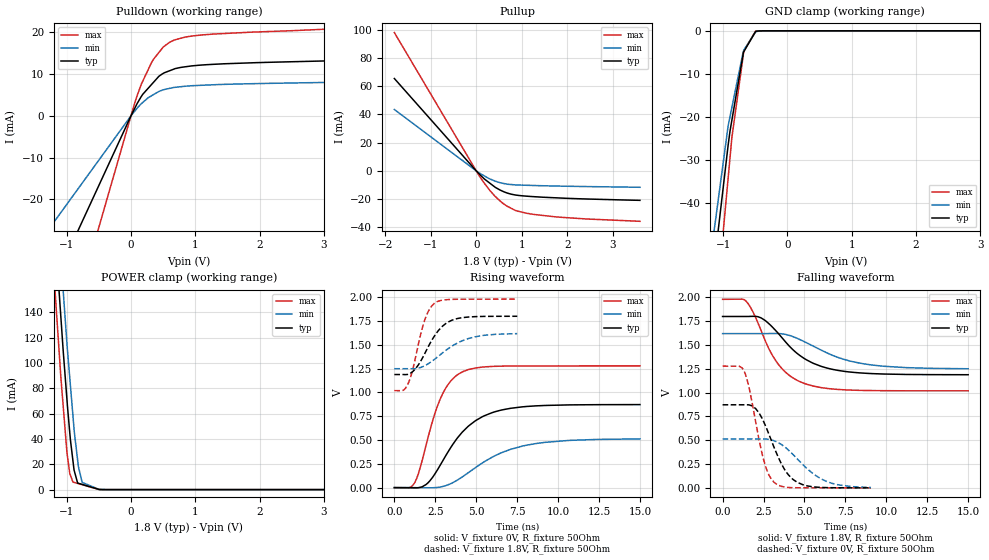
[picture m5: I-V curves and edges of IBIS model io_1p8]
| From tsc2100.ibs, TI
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|   io_1p8 Model
[Model]   io_1p8
Model_type   I/O
Polarity   Non-Inverting
Enable   Active-Low
Vinl = 0.54
Vinh = 1.26
Vmeas = 0.9
Vref = 0.9
Cref = 10pF
Rref = 50
|   typ   min   max
|   (nom PVT)   (fast PVT)   (slow PVT)
|C_comp from frequency sweep method (F=13MHz)
|Average
|C_comp   3.038e-12   2.861e-12   3.135e-12
|ON state : BUFFER OUTPUT TURNED HIGH
|C_comp   4.296e-12   3.958e-12   4.472e-12
|OFF state: BUFFER IN HIGH IMPEDANCE
|C_comp   1.781e-12   1.764e-12   1.798e-12
|C_comp from LC tank measurement(L=1nH)
|Average
|Resonant Frequency(Hz)   4.230e+09   4.260e+09   4.200e+09
C_comp   1.419e-12   1.398e-12   1.440e-12
|ON state : BUFFER OUTPUT TURNED HIGH
|Resonant Frequency(Hz)   4.150e+09   4.180e+09   4.100e+09
|C_comp   1.472e-12   1.451e-12   1.508e-12
|OFF state: BUFFER IN HIGH IMPEDANCE
|Resonant Frequency(Hz)   4.310e+09   4.340e+09   4.300e+09
|C_comp   1.365e-12   1.346e-12   1.371e-12
| Where nom  PVT is Nominal Process, 1.8V, 26C
|   Fast PVT is Strong Process,  1.98V, -40C
|   Slow PVT is Weak Process,   1.62V, 86C
[Model Spec]
|Subparameter   typ   min   max
Vinh   1.26   1.134   1.386
Vinl   0.54   0.486   0.594
[Voltage Range]   1.8   1.62   1.98
|Ambient Temperature   25   85   -40
|Junction Temperature
[Temperature Range]   26   86   -40
[Pullup Reference]   1.8   1.62   1.98
[Pulldown Reference]   0   0   0
[Power Clamp Reference]   1.8   1.62   1.98
[GND Clamp Reference]   0   0   0
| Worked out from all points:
|   slope of the pulldown table from 0 to 0.27 V, typ, clamps not added: 40.6 ohm
|   slope of the pullup table from 0 to 0.27 V, typ, clamps not added: 33.6 ohm
|   GND clamp passes 1 mA (typ) near -0.53 V on its own axis
|   falling waveform, V_fixture 1.8V, R_fixture 50Ohm: 20-80 % time 2.41ns typ, 3.11ns min, 1.85ns max; typ from 1.8 V to 1.19 V
|   rising waveform, V_fixture 0V, R_fixture 50Ohm: 20-80 % time 2.33ns typ, 3.19ns min, 1.41ns max; typ from 0 V to 0.872 V
|   rising waveform, V_fixture 1.8V, R_fixture 50Ohm: 20-80 % time 1.29ns typ, 1.91ns min, 837ps max; typ from 1.19 V to 1.8 V
|   falling waveform, V_fixture 0V, R_fixture 50Ohm: 20-80 % time 1.35ns typ, 1.98ns min, 918ps max; typ from 0.872 V to 0 V
[Pulldown]
|   Voltage   I(typ)   I(min)   I(max)
-1.8V     -60.05mA   -38.22mA   -96.1mA
-72mV     -2.402mA   -1.529mA   -3.844mA
57.42mV   1.766mA    1.1mA      3.013mA
158.4mV   4.582mA    2.864mA    7.488mA
322.7mV   7.551mA    4.829mA    12.85mA
433.8mV   9.46mA     5.824mA    15.16mA
499mV     10.13mA    6.199mA    16.43mA
601.9mV   10.79mA    6.572mA    17.62mA
687.6mV   11.3mA     6.819mA    18.21mA
855.4mV   11.75mA    7.091mA    18.88mA
1.277V    12.31mA    7.423mA    19.56mA
3.6V      13.43mA    8.126mA    21.12mA
[GND Clamp]
|   Voltage   I(typ)   I(min)   I(max)
-1.8V     -235.7mA   -126.6mA   -353.2mA
-1.168V   -58.15mA   -49.61mA   -74.14mA
-923.4mV  -26.69mA   -22.19mA   -34.39mA
-892.8mV  -23.26mA   -19.91mA   -29.42mA
-863.3mV  -20.68mA   -17.74mA   -24.68mA
-693.4mV  -5.808mA   -5.249mA   -6.341mA
-684mV    -4.989mA   -4.788mA   -5.33mA
-677.2mV  -4.813mA   -4.451mA   -4.592mA
-495mV    -141.9uA   -251uA     -60.12uA
-315.9mV  -1.107uA   -2.785uA   -80.72nA
3.6V      0A         0A         0A
[Pullup]
|   Voltage   I(typ)   I(min)   I(max)
-1.8V     65.5mA     43.52mA    98.09mA
71.28mV   -2.408mA   -1.592mA   -3.711mA
180mV     -5.804mA   -3.627mA   -8.846mA
348.5mV   -9.964mA   -6.401mA   -15.74mA
601.9mV   -14.79mA   -8.961mA   -23.42mA
889mV     -17.28mA   -10.02mA   -28.39mA
1.277V    -18.36mA   -10.42mA   -30.98mA
2.376V    -19.94mA   -11.15mA   -34.07mA
3.6V      -20.95mA   -11.67mA   -35.81mA
[POWER Clamp]
|   Voltage   I(typ)   I(min)   I(max)
-1.8V     694.4mA    728.5mA    661.7mA
-1.22V    231.8mA    280.1mA    186.8mA
-1.136V   169.5mA    214.6mA    122.7mA
-1.091V   136.6mA    182.9mA    88.99mA
-1.055V   110mA      157.2mA    66.24mA
-994mV    69.75mA    114.1mA    28.51mA
-952.4mV  45.19mA    88.52mA    12.85mA
-902.9mV  22.79mA    58.45mA    5.938mA
-818.1mV  4.984mA    18.28mA    4.715mA
-759.8mV  4.103mA    5.698mA    3.874mA
-494.1mV  100.5uA    125.2uA    53.01uA
3.6V      0A         0A         0A
[Ramp]
R_load = 50
|   typ   min   max
dV/dt_r   0.523306/2.32414e-09   0.30704/3.17186e-09   0.76723/1.40904e-09
dV/dt_f   0.367029/2.40592e-09   0.221392/3.0976e-09   0.576578/1.84684e-09
[Falling Waveform]
V_fixture = 1.8V
V_fixture_min = 1.62V
V_fixture_max = 1.98V
R_fixture = 50Ohm
|   Time   V(typ)   V(min)   V(max)
0s        1.8V       1.62V      1.98V
1.448ns   1.8V       1.62V      1.959V
1.847ns   1.802V     1.62V      1.851V
2.348ns   1.786V     1.62V      1.655V
3.286ns   1.644V     1.621V     1.326V
4.024ns   1.498V     1.604V     1.189V
4.963ns   1.362V     1.538V     1.099V
6.36ns    1.259V     1.419V     1.045V
8.376ns   1.208V     1.31V      1.024V
15ns      1.188V     1.251V     1.019V
[Rising Waveform]
V_fixture = 0V
V_fixture_min = 0V
V_fixture_max = 0V
R_fixture = 50Ohm
|   Time   V(typ)   V(min)   V(max)
0s        1.048nV    7.733nV    577pV
1.233ns   -2.484mV   -98.86uV   48.19mV
1.507ns   204.9uV    -757.5uV   167.5mV
2.047ns   48.95mV    -1.909mV   518.8mV
2.805ns   236.9mV    6.393mV    931.8mV
3.403ns   409.3mV    38.26mV    1.11V
4.143ns   581.4mV    111.6mV    1.215V
5.487ns   754mV      271.3mV    1.268V
7.983ns   850.9mV    442.3mV    1.278V
15ns      872.2mV    511.7mV    1.279V
[Rising Waveform]
V_fixture = 1.8V
V_fixture_min = 1.62V
V_fixture_max = 1.98V
R_fixture = 50Ohm
|   Time   V(typ)   V(min)   V(max)
0s        1.188V     1.249V     1.019V
535ps     1.188V     1.249V     1.022V
819ps     1.189V     1.249V     1.084V
1.096ns   1.215V     1.248V     1.222V
1.818ns   1.395V     1.277V     1.741V
2.447ns   1.592V     1.347V     1.936V
3.141ns   1.723V     1.441V     1.973V
3.822ns   1.775V     1.516V     1.979V
5.341ns   1.798V     1.596V     1.98V
7.508ns   1.8V       1.618V     1.98V
[Falling Waveform]
V_fixture = 0V
V_fixture_min = 0V
V_fixture_max = 0V
R_fixture = 50Ohm
|   Time   V(typ)   V(min)   V(max)
0s        872.5mV    513.8mV    1.279V
1.326ns   872.5mV    513.9mV    1.223V
1.631ns   871mV      513.9mV    1.043V
2.015ns   833.5mV    513.8mV    699.2mV
2.512ns   694.5mV    513.8mV    292.5mV
3.204ns   400.9mV    490.9mV    50.29mV
4.02ns    137mV      397.7mV    3.811mV
4.898ns   33.54mV    245.3mV    979.3uV
6.51ns    2.133mV    57.34mV    368.7uV
9.064ns   253.3uV    3.852mV    119.5uV
